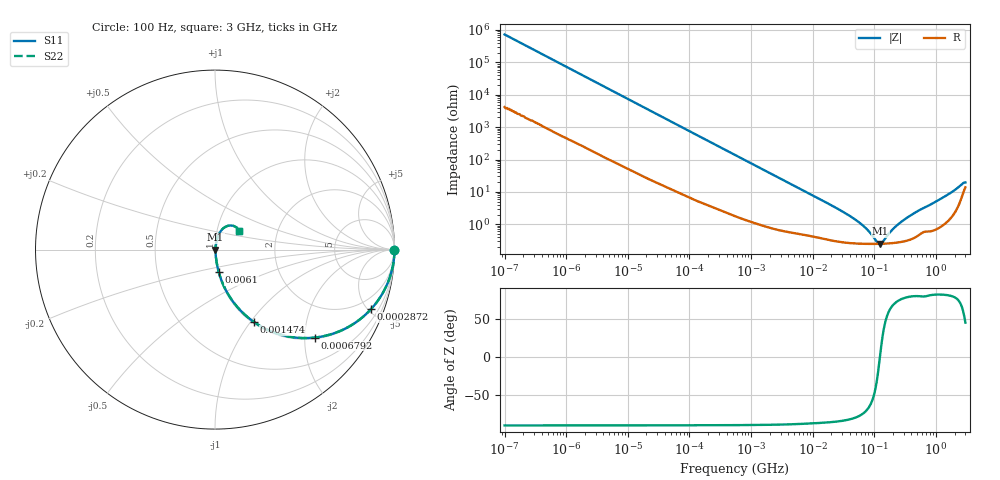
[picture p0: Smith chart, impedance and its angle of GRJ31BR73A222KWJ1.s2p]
!Murata Part Number: GRJ31BR73A222KWJ1
!These Parameters are Measured in Series Mode Connection
!Data Generated on Jun 19, 2026
!  o--ll--o
!Port1  Port2
!  o------o
!Operation Temp=25[degC], DC Bias Voltage=0[V]
!Freq. Start=100[Hz] Stop=3[GHz] 401[Steps]
# Hz S RI R 50
!Freq.(Hz) S11(Real) S11(Imag) S21(Real) S21(Imag) S12(Real) S12(Imag) S22(Real) S22(Imag)
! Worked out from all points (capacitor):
!   401 points, 100 Hz to 3 GHz, reference 50 ohm
!   read as one part in series: C = 2.18 nF near 109 Hz
!   lowest |Z| = 249 mohm at 124.1 MHz (marker M1)
!   series resonance near 123 MHz, so ESL is about 770 pH
!   S11 on the Smith chart (normalised r, x): 100 Hz: open; 287.2 kHz: 1.06, -5.25; 679.2 kHz: 1.03, -2.23; 1.474 MHz: 1.02, -1.04; 6.1 MHz: 1.01, -0.25; 3 GHz: 1.28, +0.28
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100  1 -0.000137  8e-07 0.000137  8e-07 0.000137  1 -0.000137
1788  1 -0.00243  2.15e-05 0.00243  2.15e-05 0.00243  1 -0.00243
31977  0.9978 -0.0428  0.00216 0.0428  0.00216 0.0428  0.9978 -0.0428
106717  0.979 -0.1391  0.021 0.1391  0.021 0.1391  0.979 -0.1391
287190  0.8707 -0.33  0.1293 0.33  0.1293 0.33  0.8707 -0.33
547723  0.6549 -0.469  0.3451 0.469  0.3451 0.469  0.6549 -0.469
679242  0.5544 -0.4903  0.4456 0.4903  0.4456 0.4903  0.5544 -0.4903
1473992  0.2155 -0.4023  0.7845 0.4023  0.7845 0.4023  0.2155 -0.4023
2692740  0.0802 -0.26  0.9198 0.26  0.9198 0.26  0.0802 -0.26
6100390  0.0205 -0.1232  0.9795 0.1232  0.9795 0.1232  0.0205 -0.1232
9794414  0.0103 -0.078  0.9897 0.078  0.9897 0.078  0.0103 -0.078
5.026954e7  0.00271 -0.0132  0.9973 0.0132  0.9973 0.0132  0.00271 -0.0132
7.405258e7  0.00252 -0.00685  0.9975 0.00685  0.9975 0.00685  0.00252 -0.00685
1.090876e8  0.00247 -0.00156  0.9975 0.00156  0.9975 0.00156  0.00247 -0.00156
1.241234e8  0.00248 0.000116  0.9975 -0.000116  0.9975 -0.000116  0.00248 0.000116
1.412317e8  0.00251 0.00179  0.9975 -0.00179  0.9975 -0.00179  0.00251 0.00179
1.751444e8  0.00259 0.00467  0.9974 -0.00467  0.9974 -0.00467  0.00259 0.00467
2.471375e8  0.00284 0.00979  0.9972 -0.00979  0.9972 -0.00979  0.00284 0.00979
3.800727e8  0.00365 0.0179  0.9964 -0.0179  0.9964 -0.0179  0.00365 0.0179
1.789813e9  0.025 0.0922  0.975 -0.0922  0.975 -0.0922  0.025 0.0922
2.636591e9  0.0862 0.1347  0.9138 -0.1347  0.9138 -0.1347  0.0862 0.1347
3e9  0.134 0.1062  0.866 -0.1062  0.866 -0.1062  0.134 0.1062
